| TEXAS INSTRUMENTS INCORPORATED
| Standard Linear and Logic Group
| IBIS Model of SN74AVC16373
| 16-BIT TRANSPARENT D-TYPE LATCH WITH 3-STATE OUTPUTS
| This file contains package information for the following:
|  TSSOP 48-pin (DGG) package as [Component] AVC16373_DGG
|  TVSOP 48-pin (DGV) package as [Component] AVC16373_DGV
| This device can be powered at the following Vccs:
|  1.2 volt Vcc
|  1.5 volt Vcc
|  1.8 volt Vcc
|  2.5 volt Vcc
|  3.3 volt Vcc
| This file provides unique models under the [Model Selector] for each Vcc.
| For operation at a specific Vcc, select the appropriate model after each
| [Model Selector] keyword.
[IBIS Ver]   3.2
[Comment char]  |_char
[File Name]   sn74avc16373.ibs
[File Rev]   1.1 | x_die
[Date]   February 10, 2004
[Source]   Data created from TI-SPICE simulations at TI-SLL.
[Notes]   The following is an IBIS list for the AVC16373.
   Please contact sllibis@ti.com with questions and
   comments concerning SLL IBIS models.
   - FILE REV HISTORY
   - 1.1 Release IBIS file on 02/10/04
   - Power clamp data deleted as there is no power-clamp diode.
   - IBIS 3.2 SYNTAX CANNOT DESCRIBE THE CHARACTERISTICS OF
   ANY OUTPUT STRUCTURES THAT DYNAMICALLY CHANGES THE
   IMPEDANCES DURING THE TRANSITION. THIS DEVICE USE SIMILAR
   OUTPUT STRUCTURE AND THEREFORE THE SIMULATION RESULTS
   MAY NOT BE ACCURATE. TI RECOMMENDS THE USE OF SPICE
   SIMULATION WHEN SIMULATION ACCURACY IS IMPORTANT.
[Disclaimer] Property of Texas Instruments Incorporated.  Unauthorized
   reproduction and/or distribution is strictly prohibited.
   This product is protected under copyright law.
   Created  2004, (C) Copyright  2004, Texas Instruments
   Incorporated, All Rights Reserved
   UNLESS THERE IS A SIGNED, WRITTEN AGREEMENT TO THE
   CONTRARY, TEXAS INSTRUMENTS (TI) IS PROVIDING THE IBIS
   MODELS  AND WITHOUT ANY WARRANTY, EXPRESSED OR
   IMPLIED.  TI assumes no liability for:
   1) the accuracy of the IBIS models provided to your
   company;
   2) the proper functioning of these IBIS Models in your
   design or for any resulting applications; or
   3) infringement of patents, copyrights or intellectual
   property rights resulting from your use of these IBIS
   models.
   TI provides IBIS Models as a service to our customers.
   You and your company shall not distribute, sell or give
   these models to anyone else without prior written
   permission from TI.
   TI reserves the right to make changes to our products or
   to discontinue any semiconductor product or service
   without notice, and advises our customers to obtain the
   latest version of relevant information to verify, before
   placing orders, that the information being relied on is
   current.
   Please be aware that your receipt and use of the IBIS
   information provided shall serve as acceptance of these
   terms and conditions.  If you do not accept these terms,
   you should return or destroy the IBIS models and any
   other accompanying information immediately.
| Component AVC16373_DGG 48-pin TSSOP
[Component]   AVC16373_DGG
[Manufacturer]   Texas Instruments, Inc.
[Package]
|   typ   min   max
R_pkg   4.400e-02   3.800e-02   5.100e-02
L_pkg   3.019e-09   2.486e-09   4.099e-09
C_pkg   5.070e-13   3.340e-13   8.090e-13
[Pin]   signal_name   model_name   R_pin   L_pin   C_pin
1   1OE   AVC16373_NOE   4.100e-02   4.017e-09   7.590e-13
2   1Q1   AVC16373_OUT   4.200e-02   3.737e-09   7.920e-13
3   1Q2   AVC16373_OUT   4.200e-02   3.480e-09   6.610e-13
4   GND   GND   3.800e-02   3.131e-09   5.750e-13
5   1Q3   AVC16373_OUT   4.700e-02   3.122e-09   5.660e-13
6   1Q4   AVC16373_OUT   4.300e-02   2.948e-09   5.040e-13
7   VCC   POWER   4.500e-02   2.845e-09   3.970e-13
8   1Q5   AVC16373_OUT   4.900e-02   2.835e-09   3.940e-13
9   1Q6   AVC16373_OUT   4.800e-02   2.715e-09   3.780e-13
10   GND   GND   5.000e-02   2.664e-09   3.630e-13
11   1Q7   AVC16373_OUT   5.000e-02   2.585e-09   3.480e-13
12   1Q8   AVC16373_OUT   4.900e-02   2.550e-09   3.370e-13
13   2Q1   AVC16373_OUT   4.900e-02   2.541e-09   3.360e-13
14   2Q2   AVC16373_OUT   5.000e-02   2.574e-09   3.480e-13
15   GND   GND   4.900e-02   2.618e-09   3.590e-13
16   2Q3   AVC16373_OUT   4.600e-02   2.671e-09   3.750e-13
17   2Q4   AVC16373_OUT   4.500e-02   2.754e-09   3.890e-13
18   VCC   POWER   4.400e-02   2.823e-09   4.500e-13
19   2Q5   AVC16373_OUT   4.200e-02   2.968e-09   5.030e-13
20   2Q6   AVC16373_OUT   5.100e-02   3.108e-09   5.350e-13
21   GND   GND   4.200e-02   3.175e-09   5.870e-13
22   2Q7   AVC16373_OUT   4.100e-02   3.449e-09   6.780e-13
23   2Q8   AVC16373_OUT   4.400e-02   3.766e-09   8.040e-13
24   2OE   AVC16373_NOE   4.300e-02   4.065e-09   7.610e-13
25   2LE   AVC16373_LE   4.100e-02   3.994e-09   7.570e-13
26   2D8   AVC16373_IN   3.900e-02   3.649e-09   7.890e-13
27   2D7   AVC16373_IN   3.800e-02   3.362e-09   6.600e-13
28   GND   GND   3.800e-02   3.082e-09   5.740e-13
29   2D6   AVC16373_IN   4.400e-02   2.990e-09   5.220e-13
30   2D5   AVC16373_IN   4.100e-02   2.917e-09   4.950e-13
31   VCC   POWER   4.300e-02   2.820e-09   4.480e-13
32   2D4   AVC16373_IN   4.300e-02   2.699e-09   3.850e-13
33   2D3   AVC16373_IN   4.500e-02   2.628e-09   3.720e-13
34   GND   GND   4.600e-02   2.556e-09   3.560e-13
35   2D2   AVC16373_IN   4.600e-02   2.495e-09   3.440e-13
36   2D1   AVC16373_IN   4.700e-02   2.487e-09   3.340e-13
37   1D8   AVC16373_IN   4.700e-02   2.490e-09   3.350e-13
38   1D7   AVC16373_IN   4.600e-02   2.486e-09   3.430e-13
39   GND   GND   4.500e-02   2.566e-09   3.560e-13
40   1D6   AVC16373_IN   4.400e-02   2.639e-09   3.740e-13
41   1D5   AVC16373_IN   4.300e-02   2.701e-09   3.860e-13
42   VCC   POWER   4.300e-02   2.817e-09   4.500e-13
43   1D4   AVC16373_IN   4.100e-02   2.935e-09   5.010e-13
44   1D3   AVC16373_IN   4.700e-02   3.035e-09   5.290e-13
45   GND   GND   4.300e-02   3.171e-09   5.890e-13
46   1D2   AVC16373_IN   4.000e-02   3.415e-09   6.820e-13
47   1D1   AVC16373_IN   4.300e-02   3.741e-09   8.090e-13
48   1LE   AVC16373_LE   4.400e-02   4.099e-09   7.640e-13
| Component AVC16373_DGV 48-pin TVSOP
[Component]   AVC16373_DGV
[Manufacturer]   Texas Instruments, Inc.
[Package]
|   typ   min   max
R_pkg   7.000e-02   4.900e-02   8.500e-02
L_pkg   3.013e-09   2.743e-09   3.408e-09
C_pkg   3.710e-13   2.940e-13   5.110e-13
[Pin]   signal_name   model_name   R_pin   L_pin   C_pin
1   1OE   AVC16373_NOE   4.900e-02   3.393e-09   4.970e-13
2   1Q1   AVC16373_OUT   6.000e-02   3.250e-09   5.020e-13
3   1Q2   AVC16373_OUT   7.700e-02   3.310e-09   4.510e-13
4   GND   GND   8.500e-02   3.299e-09   4.040e-13
5   1Q3   AVC16373_OUT   8.300e-02   3.136e-09   3.600e-13
6   1Q4   AVC16373_OUT   7.700e-02   3.019e-09   3.630e-13
7   VCC   POWER   6.500e-02   2.882e-09   3.490e-13
8   1Q5   AVC16373_OUT   6.600e-02   2.829e-09   3.140e-13
9   1Q6   AVC16373_OUT   6.700e-02   2.796e-09   3.140e-13
10   GND   GND   6.900e-02   2.754e-09   3.080e-13
11   1Q7   AVC16373_OUT   7.000e-02   2.753e-09   3.010e-13
12   1Q8   AVC16373_OUT   7.100e-02   2.745e-09   2.940e-13
13   2Q1   AVC16373_OUT   7.000e-02   2.744e-09   2.940e-13
14   2Q2   AVC16373_OUT   7.000e-02   2.754e-09   3.010e-13
15   GND   GND   6.900e-02   2.754e-09   3.080e-13
16   2Q3   AVC16373_OUT   6.700e-02   2.796e-09   3.140e-13
17   2Q4   AVC16373_OUT   6.600e-02   2.829e-09   3.140e-13
18   VCC   POWER   6.500e-02   2.883e-09   3.500e-13
19   2Q5   AVC16373_OUT   7.500e-02   3.014e-09   3.630e-13
20   2Q6   AVC16373_OUT   8.000e-02   3.128e-09   3.580e-13
21   GND   GND   8.400e-02   3.295e-09   4.030e-13
22   2Q7   AVC16373_OUT   7.800e-02   3.311e-09   4.520e-13
23   2Q8   AVC16373_OUT   6.200e-02   3.259e-09   5.010e-13
24   2OE   AVC16373_NOE   5.200e-02   3.404e-09   4.960e-13
25   2LE   AVC16373_LE   5.300e-02   3.397e-09   5.050e-13
26   2D8   AVC16373_IN   6.200e-02   3.249e-09   5.110e-13
27   2D7   AVC16373_IN   7.700e-02   3.308e-09   4.530e-13
28   GND   GND   8.200e-02   3.289e-09   4.030e-13
29   2D6   AVC16373_IN   7.800e-02   3.121e-09   3.590e-13
30   2D5   AVC16373_IN   7.400e-02   3.010e-09   3.630e-13
31   VCC   POWER   6.500e-02   2.883e-09   3.490e-13
32   2D4   AVC16373_IN   6.700e-02   2.829e-09   3.140e-13
33   2D3   AVC16373_IN   6.700e-02   2.795e-09   3.140e-13
34   GND   GND   6.900e-02   2.753e-09   3.070e-13
35   2D2   AVC16373_IN   7.000e-02   2.753e-09   3.010e-13
36   2D1   AVC16373_IN   7.000e-02   2.743e-09   2.940e-13
37   1D8   AVC16373_IN   7.000e-02   2.743e-09   2.940e-13
38   1D7   AVC16373_IN   7.000e-02   2.753e-09   3.010e-13
39   GND   GND   6.900e-02   2.754e-09   3.070e-13
40   1D6   AVC16373_IN   6.800e-02   2.797e-09   3.140e-13
41   1D5   AVC16373_IN   6.700e-02   2.830e-09   3.140e-13
42   VCC   POWER   6.400e-02   2.880e-09   3.490e-13
43   1D4   AVC16373_IN   7.200e-02   3.004e-09   3.620e-13
44   1D3   AVC16373_IN   7.800e-02   3.121e-09   3.590e-13
45   GND   GND   8.400e-02   3.296e-09   4.030e-13
46   1D2   AVC16373_IN   7.700e-02   3.308e-09   4.510e-13
47   1D1   AVC16373_IN   6.200e-02   3.258e-09   4.990e-13
48   1LE   AVC16373_LE   5.300e-02   3.408e-09   4.940e-13
| Model AVC16373_IN
[Model Selector]   AVC16373_IN
AVC16373_IN_12   1.2 volt Vcc
AVC16373_IN_15   1.5 volt Vcc
AVC16373_IN_18   1.8 volt Vcc
AVC16373_IN_25   2.5 volt Vcc
AVC16373_IN_33   3.3 volt Vcc
| Model AVC16373_NOE
[Model Selector]   AVC16373_NOE
AVC16373_NOE_12   1.2 volt Vcc
AVC16373_NOE_15   1.5 volt Vcc
AVC16373_NOE_18   1.8 volt Vcc
AVC16373_NOE_25   2.5 volt Vcc
AVC16373_NOE_33   3.3 volt Vcc
| Model AVC16373_LE
[Model Selector]   AVC16373_LE
AVC16373_LE_12   1.2 volt Vcc
AVC16373_LE_15   1.5 volt Vcc
AVC16373_LE_18   1.8 volt Vcc
AVC16373_LE_25   2.5 volt Vcc
AVC16373_LE_33   3.3 volt Vcc
| Model AVC16373_OUT
[Model Selector]   AVC16373_OUT
AVC16373_OUT_12   1.2 volt Vcc
AVC16373_OUT_15   1.5 volt Vcc
AVC16373_OUT_18   1.8 volt Vcc
AVC16373_OUT_25   2.5 volt Vcc
AVC16373_OUT_33   3.3 volt Vcc
| Models and submodels in the file (20): AVC16373_IN_12 (Input), AVC16373_IN_15 (Input), AVC16373_IN_18 (Input), AVC16373_IN_25 (Input), AVC16373_IN_33 (Input), AVC16373_NOE_12 (Input), AVC16373_NOE_15 (Input), AVC16373_NOE_18 (Input), AVC16373_NOE_25 (Input), AVC16373_NOE_33 (Input), AVC16373_LE_12 (Input), AVC16373_LE_15 (Input), AVC16373_LE_18 (Input), AVC16373_LE_25 (Input), AVC16373_LE_33 (Input), AVC16373_OUT_12 (3-state), AVC16373_OUT_15 (3-state), AVC16373_OUT_18 (3-state), AVC16373_OUT_25 (3-state), AVC16373_OUT_33 (3-state)
